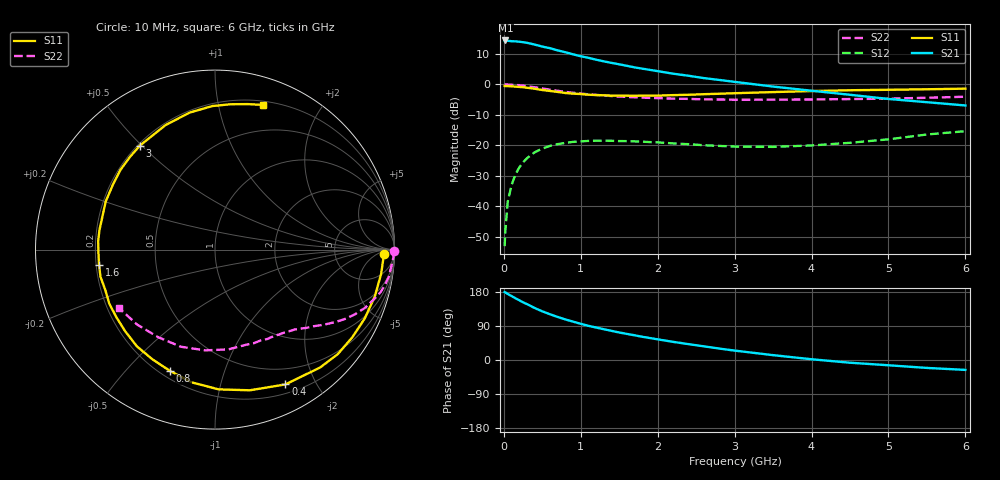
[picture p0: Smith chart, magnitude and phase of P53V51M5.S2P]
! SIEMENS Small Signal Semiconductors
! BFP183
! Si NPN RF Bipolar Junction Transistor in SOT143
! VCE = 3.5 V  IC = 1.5 mA
! Common Emitter S-Parameters:  March  1996
# GHz  S  MA  R  50
!  f  S11  S21  S12  S22
! GHz  MAG  ANG  MAG  ANG  MAG  ANG  MAG  ANG
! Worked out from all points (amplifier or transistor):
!   36 points, 10 MHz to 6 GHz, reference 50 ohm
!   highest |S21| = 14.4 dB at 20 MHz (marker M1)
!   |S21| within 3 dB of that: start of sweep to 662.9 MHz
!   unconditionally stable (mu >= 1): 2.274 GHz to 5.934 GHz
!   at 250 MHz: K = 0.11, MSG = 19.7 dB, |S12| = -25.6 dB
!   at 1.4 GHz: K = 0.60, MSG = 12.8 dB, |S12| = -18.5 dB
!   at 6 GHz: K = 0.99, MSG = 4.2 dB, |S12| = -15.4 dB
!   S11 on the Smith chart (normalised r, x): 10 MHz: 27, -13; 400 MHz: 0.30, -1.61; 800 MHz: 0.24, -0.67; 1.6 GHz: 0.21, -0.06; 3 GHz: 0.21, +0.49; 6 GHz: 0.23, +1.36
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0.01  0.9411 -1.6  5.208 179.2  0.0022 82.4  0.9995 -0.6
0.02  0.9387 -3.4  5.259 178.3  0.004 83.4  0.9978 -1.2
0.05  0.9355 -8.3  5.201 174.3  0.0117 87.2  0.9935 -3.0
0.1  0.9279 -16.3  5.111 168.8  0.0221 81.0  0.9856 -6.0
0.15  0.9183 -24.7  5.085 163.1  0.033 75.3  0.9795 -9.0
0.25  0.8983 -40.5  4.915 152.2  0.0524 66.7  0.9528 -14.4
0.3  0.88 -48.3  4.818 147.5  0.0611 62.4  0.9328 -16.8
0.4  0.8473 -62.4  4.504 137.3  0.0765 54.7  0.8958 -21.3
0.5  0.8075 -76.1  4.174 128.4  0.088 47.6  0.8558 -25.1
0.6  0.779 -88.5  3.923 120.7  0.0976 41.2  0.8182 -28.3
0.8  0.7212 -110.2  3.371 107.0  0.1092 31.4  0.7528 -33.3
0.9  0.7038 -119.7  3.115 101.2  0.1135 27.5  0.7276 -35.3
1.1  0.6761 -137.8  2.724 90.1  0.1178 20.8  0.6857 -38.8
1.3  0.6616 -152.9  2.386 81.2  0.1189 15.0  0.6559 -42.0
1.6  0.6515 -172.6  2.014 68.8  0.1168 9.2  0.6222 -46.3
1.9  0.6529 170.5  1.727 57.9  0.1126 5.4  0.5993 -50.9
2.2  0.6654 156.2  1.496 47.9  0.1072 3.5  0.5823 -56.0
3  0.7148 125.8  1.099 24.8  0.095 6.1  0.5582 -71.4
3.5  0.7464 111.7  0.919 12.8  0.094 12.0  0.5608 -82.3
4.5  0.8001 91.0  0.674 -7.2  0.1097 22.7  0.5737 -109.4
5.5  0.8306 77.4  0.509 -20.9  0.1502 25.3  0.6022 -136.1
6  0.85 71.5  0.45 -26.1  0.1702 22.1  0.6263 -148.7
